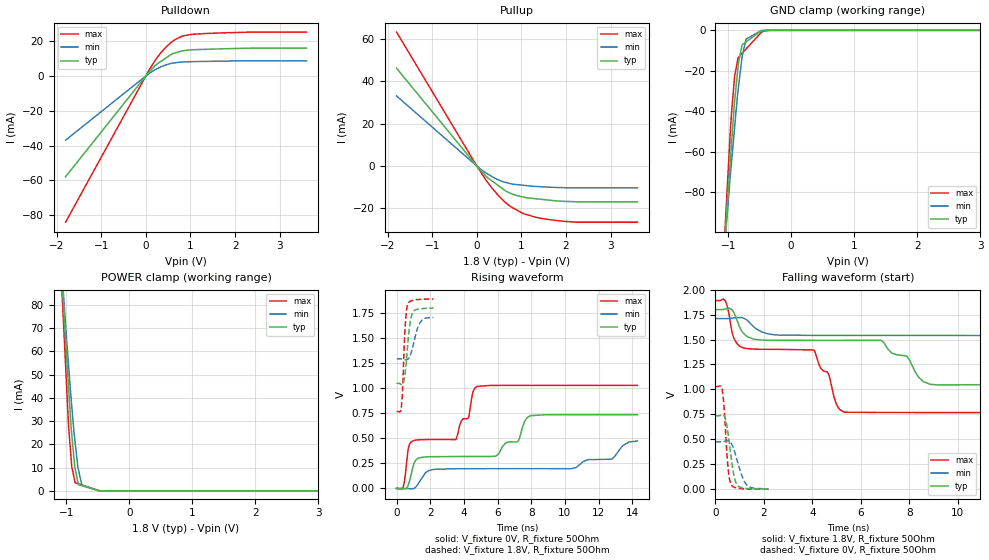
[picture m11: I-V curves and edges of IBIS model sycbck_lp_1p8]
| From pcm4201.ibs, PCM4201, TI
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|   sycbck_lp_1p8 Model
[Model]   sycbck_lp_1p8
Model_type   I/O
Polarity   Non-Inverting
Enable   Active-Low
Vinl = 0.54
Vinh = 1.26
Vmeas = 0.9
Vref = 0.9
Cref = 2pF
Rref = 50
|   typ   min   max
|   (nom PVT)   (fast PVT)   (slow PVT)
|C_comp from frequency sweep method (F=6.94MHz)
C_comp   1.338e-12   1.179e-12   1.504e-12
|ON state : BUFFER OUTPUT TURNED HIGH
|C_comp   1.510e-12   1.305e-12   1.739e-12
|OFF state: BUFFER IN HIGH IMPEDANCE
|C_comp   1.338e-12   1.179e-12   1.504e-12
|C_comp from LC tank measurement(L=1nH)
|Average
|Resonant Frequency(Hz)   7.410e+09   7.675e+09   7.155e+09
|C_comp   4.618e-13   4.304e-13   4.953e-13
|ON state : BUFFER OUTPUT TURNED HIGH
|Resonant Frequency(Hz)   7.400e+09   7.640e+09   7.170e+09
|C_comp   4.630e-13   4.344e-13   4.932e-13
|OFF state: BUFFER IN HIGH IMPEDANCE
|Resonant Frequency(Hz)   7.420e+09   7.710e+09   7.140e+09
|C_comp   4.605e-13   4.265e-13   4.974e-13
| Where nom  PVT is Nominal Process, 1.8V, 35C
|   Fast PVT is Strong Process,  1.89V, -10C
|   Slow PVT is Weak Process,   1.71V, 80C
[Model Spec]
Vinl   0.54   0.513   0.567
Vinh   1.26   1.197   1.323
[Voltage Range]   1.8   1.71   1.89
|Ambient Temperature   25   70   -10
|Junction Temperature
[Temperature Range]   35   80   -10
[Pullup Reference]   1.8   1.71   1.89
[Pulldown Reference]   0   0   0
[Power Clamp Reference]   1.8   1.71   1.89
[GND Clamp Reference]   0   0   0
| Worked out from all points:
|   slope of the pulldown table from 0 to 0.27 V, typ, clamps not added: 37.4 ohm
|   slope of the pullup table from 0 to 0.27 V, typ, clamps not added: 45.3 ohm
|   GND clamp passes 1 mA (typ) near -0.51 V on its own axis
|   falling waveform, V_fixture 1.8V, R_fixture 50Ohm: 20-80 % time 7.25ns typ, 12.9ns min, 4.22ns max; typ from 1.8 V to 1.05 V
|   rising waveform, V_fixture 0V, R_fixture 50Ohm: 20-80 % time 6.57ns typ, 11.7ns min, 3.83ns max; typ from 0 V to 0.736 V
|   rising waveform, V_fixture 1.8V, R_fixture 50Ohm: 20-80 % time 256ps typ, 400ps min, 171ps max; typ from 1.05 V to 1.8 V
|   falling waveform, V_fixture 0V, R_fixture 50Ohm: 20-80 % time 252ps typ, 372ps min, 167ps max; typ from 0.736 V to 0.002 V
[Pulldown]
|   Voltage   I(typ)   I(min)   I(max)
-1.8V     -57.89mA   -36.89mA   -83.98mA
75.6mV    2.32mA     1.436mA    3.522mA
226.8mV   6.318mA    3.809mA    9.639mA
332.6mV   8.293mA    5.198mA    13.23mA
440.4mV   10.15mA    6.265mA    16.32mA
574.6mV   12.46mA    7.222mA    19.42mA
663.4mV   13.26mA    7.557mA    21.02mA
825.9mV   14.46mA    7.994mA    22.96mA
1.058V    15.03mA    8.196mA    23.95mA
2.366V    15.95mA    8.681mA    25.18mA
3.6V      15.95mA    8.681mA    25.18mA
[GND Clamp]
|   Voltage   I(typ)   I(min)   I(max)
-1.8V     -506.3mA   -422.2mA   -629.4mA
-1.051V   -104.7mA   -105.9mA   -99.82mA
-1.015V   -86.71mA   -91.79mA   -79.1mA
-969.6mV  -66.65mA   -73.72mA   -52.58mA
-950.7mV  -58.34mA   -67.11mA   -43.19mA
-895.9mV  -34.76mA   -47.95mA   -22.49mA
-837mV    -16.38mA   -28.49mA   -13.39mA
-777.6mV  -7.171mA   -13.18mA   -11.37mA
-716.5mV  -5.777mA   -4.369mA   -9.286mA
-470.6mV  -190uA     -45.19uA   -906.7uA
-357.2mV  -9.976uA   -3.626uA   -60.98uA
3.6V      0A         0A         0A
[Pullup]
|   Voltage   I(typ)   I(min)   I(max)
-1.8V     46.08mA    33mA       63.1mA
20.08fV   -9.81pA    -7.712pA   -13.6pA
213.6mV   -4.889mA   -3.416mA   -6.898mA
485.7mV   -9.281mA   -6.558mA   -14mA
657mV     -11.91mA   -7.795mA   -17.47mA
752.2mV   -12.84mA   -8.313mA   -19.06mA
1.058V    -14.7mA    -9.111mA   -22.54mA
1.382V    -15.55mA   -9.689mA   -24.41mA
1.784V    -16.44mA   -10.09mA   -25.67mA
2.268V    -16.87mA   -10.31mA   -26.46mA
3.6V      -16.87mA   -10.31mA   -26.46mA
[POWER Clamp]
|   Voltage   I(typ)   I(min)   I(max)
-1.8V     485.5mA    403.7mA    605.4mA
-1.062V   89.95mA    92.35mA    83.52mA
-1.033V   75.38mA    80.96mA    67.43mA
-963.9mV  45.55mA    54.71mA    28.98mA
-923.4mV  28.12mA    40.32mA    14.72mA
-911mV    24.26mA    36.39mA    10.47mA
-862.2mV  10.1mA     22.02mA    4.108mA
-812.3mV  3.643mA    9.925mA    3.148mA
-804.6mV  2.654mA    9.001mA    3.077mA
-750.7mV  2.225mA    2.486mA    2.582mA
-470.3mV  3.961uA    2.627uA    8.482uA
3.6V      0A         0A         0A
[Ramp]
R_load = 50
|   typ   min   max
dV/dt_r   0.441654/6.56557e-09   0.284902/1.17403e-08   0.617078/3.82869e-09
dV/dt_f   0.450589/7.24618e-09   0.250182/1.29318e-08   0.672895/4.2138e-09
[Falling Waveform]
V_fixture = 1.8V
V_fixture_min = 1.71V
V_fixture_max = 1.89V
R_fixture = 50Ohm
|   Time   V(typ)   V(min)   V(max)
0s        1.8V       1.71V      1.89V
400ps     1.805V     1.71V      1.889V
736ps     1.78V      1.716V     1.529V
1.064ns   1.593V     1.72V      1.425V
4.072ns   1.491V     1.541V     1.395V
5.312ns   1.491V     1.541V     772mV
6.856ns   1.489V     1.541V     768.8mV
8.872ns   1.051V     1.541V     768.5mV
12.11ns   1.049V     1.538V     768.5mV
15.99ns   1.049V     1.293V     768.5mV
[Rising Waveform]
V_fixture = 0V
V_fixture_min = 0V
V_fixture_max = 0V
R_fixture = 50Ohm
|   Time   V(typ)   V(min)   V(max)
0s        642.3pV    1.279nV    373.2pV
392ps     -2.051mV   310uV      12.04mV
816ps     102.4mV    -3.413mV   453.2mV
1.304ns   302mV      49.97mV    484.8mV
3.52ns    318.2mV    196.4mV    487.5mV
4.776ns   318.4mV    196.8mV    1.017V
7.232ns   473.3mV    197mV      1.028V
7.96ns    725.8mV    197mV      1.028V
12.78ns   736.1mV    291.6mV    1.028V
14.31ns   736.1mV    473.3mV    1.028V
[Rising Waveform]
V_fixture = 1.8V
V_fixture_min = 1.71V
V_fixture_max = 1.89V
R_fixture = 50Ohm
|   Time   V(typ)   V(min)   V(max)
0s        1.049V     1.293V     768.5mV
208ps     1.044V     1.293V     763.3mV
296ps     1.037V     1.292V     826.6mV
360ps     1.04V      1.289V     993.3mV
512ps     1.15V      1.283V     1.618V
664ps     1.432V     1.287V     1.838V
808ps     1.657V     1.326V     1.867V
976ps     1.762V     1.419V     1.877V
1.416ns   1.793V     1.659V     1.886V
2.192ns   1.799V     1.707V     1.889V
[Falling Waveform]
V_fixture = 0V
V_fixture_min = 0V
V_fixture_max = 0V
R_fixture = 50Ohm
|   Time   V(typ)   V(min)   V(max)
0s        736.1mV    475.1mV    1.028V
208ps     739.8mV    474.8mV    1.034V
288ps     745.6mV    476.7mV    979.5mV
360ps     736.9mV    479.6mV    803.9mV
512ps     573.9mV    484.9mV    230.7mV
640ps     335.4mV    464.3mV    49.94mV
776ps     124.3mV    388.1mV    20.02mV
928ps     32.96mV    261.9mV    9.632mV
1.36ns    6.082mV    27.76mV    3.215mV
2.192ns   1.68mV     2.824mV    1.013mV
